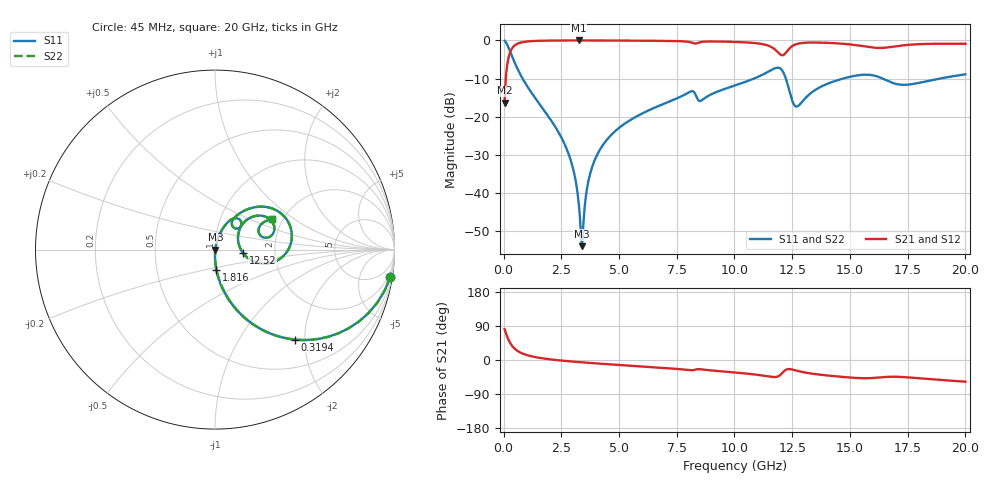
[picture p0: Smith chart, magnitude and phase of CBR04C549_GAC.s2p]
! S-parameter model data by Modelithics Inc.  support@modelithics.com 813-866-6335  Tampa FL USA
! S-Parameter data specifications:
! Substrate: 20-mil Rogers 4350B, substrate thickness, H=0.508mm, Dielectric constant, Er=3.75
! PCB Mounting Pad Footprint: Pad width, PadW=0.52mm , Pad length, PadL=0.52mm , Pad gap, PadG (edge-to-edge)=0.28mm , Reference planes=1.32mm apart
#  GHz  S  MA  R 50
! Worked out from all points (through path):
!   801 points, 45 MHz to 20 GHz, reference 50 ohm
!   highest |S21| = -0.02 dB at 3.263 GHz (marker M1); lowest = -16.3 dB at 45 MHz (marker M2)
!   group delay of S21, straight-line fit = 9.81 ps
!   lowest |S11| = -53.9 dB at 3.387 GHz (marker M3), VSWR 1.00, Z = 50.2 - j0.0323 ohm
!   |S11| at or under -10 dB: 824.3 MHz to 10.84 GHz (10.02 GHz wide, 172 % of centre); 12.22 GHz to 14.7 GHz (2.479 GHz wide, 18.4 % of centre); 16.42 GHz to 18.89 GHz (2.478 GHz wide, 14 % of centre)
!   |S22| runs from -53.9 to -0.1 dB; largest |S21 - S12| = 0
!   S11 on the Smith chart (normalised r, x): 45 MHz: 1, -13; 319.4 MHz: 0.98, -1.80; 1.816 GHz: 0.99, -0.23; 12.52 GHz: 1.37, -0.06; 20 GHz: 1.77, +0.68
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0.045  0.9883 -8.8  0.1523 81.2  0.1523 81.2  0.9883 -8.8
0.194662  0.8311 -34.1  0.5558 55.9  0.5558 55.9  0.8311 -34.1
0.319381  0.6713 -48.4  0.7407 41.6  0.7407 41.6  0.6713 -48.4
0.768369  0.3391 -71.4  0.9398 18.4  0.9398 18.4  0.3391 -71.4
1.816006  0.1143 -86.0  0.9919 3.3  0.9919 3.3  0.1143 -86.0
2.8387  0.03109 -90.0  0.9976 -3.4  0.9976 -3.4  0.03109 -90.0
3.113081  0.015 -87.4  0.9979 -4.8  0.9979 -4.8  0.015 -87.4
3.262744  0.006955 -79.0  0.9979 -5.5  0.9979 -5.5  0.006955 -79.0
3.387462  0.002017 -9.2  0.9979 -6.1  0.9979 -6.1  0.002017 -9.2
3.736675  0.0173 75.2  0.9976 -7.7  0.9976 -7.7  0.0173 75.2
4.23555  0.03982 76.8  0.9968 -9.9  0.9968 -9.9  0.03982 76.8
6.704981  0.138 68.4  0.9865 -20.0  0.9865 -20.0  0.138 68.4
10.0225  0.257 54.5  0.9547 -33.0  0.9547 -33.0  0.257 54.5
11.41935  0.3827 37.6  0.8621 -42.8  0.8621 -42.8  0.3827 37.6
11.91822  0.4373 12.2  0.6807 -42.4  0.6807 -42.4  0.4373 12.2
12.21755  0.32 -13.4  0.685 -26.1  0.685 -26.1  0.32 -13.4
12.51688  0.1581 -7.4  0.8481 -25.4  0.8481 -25.4  0.1581 -7.4
12.74137  0.1374 20.0  0.904 -29.0  0.904 -29.0  0.1374 20.0
13.36496  0.2104 42.9  0.9375 -36.1  0.9375 -36.1  0.2104 42.9
15.36046  0.3495 28.9  0.8586 -47.6  0.8586 -47.6  0.3495 28.9
16.68248  0.2909 13.0  0.8122 -44.3  0.8122 -44.3  0.2909 13.0
20  0.3596 27.8  0.9019 -57.2  0.9019 -57.2  0.3596 27.8
